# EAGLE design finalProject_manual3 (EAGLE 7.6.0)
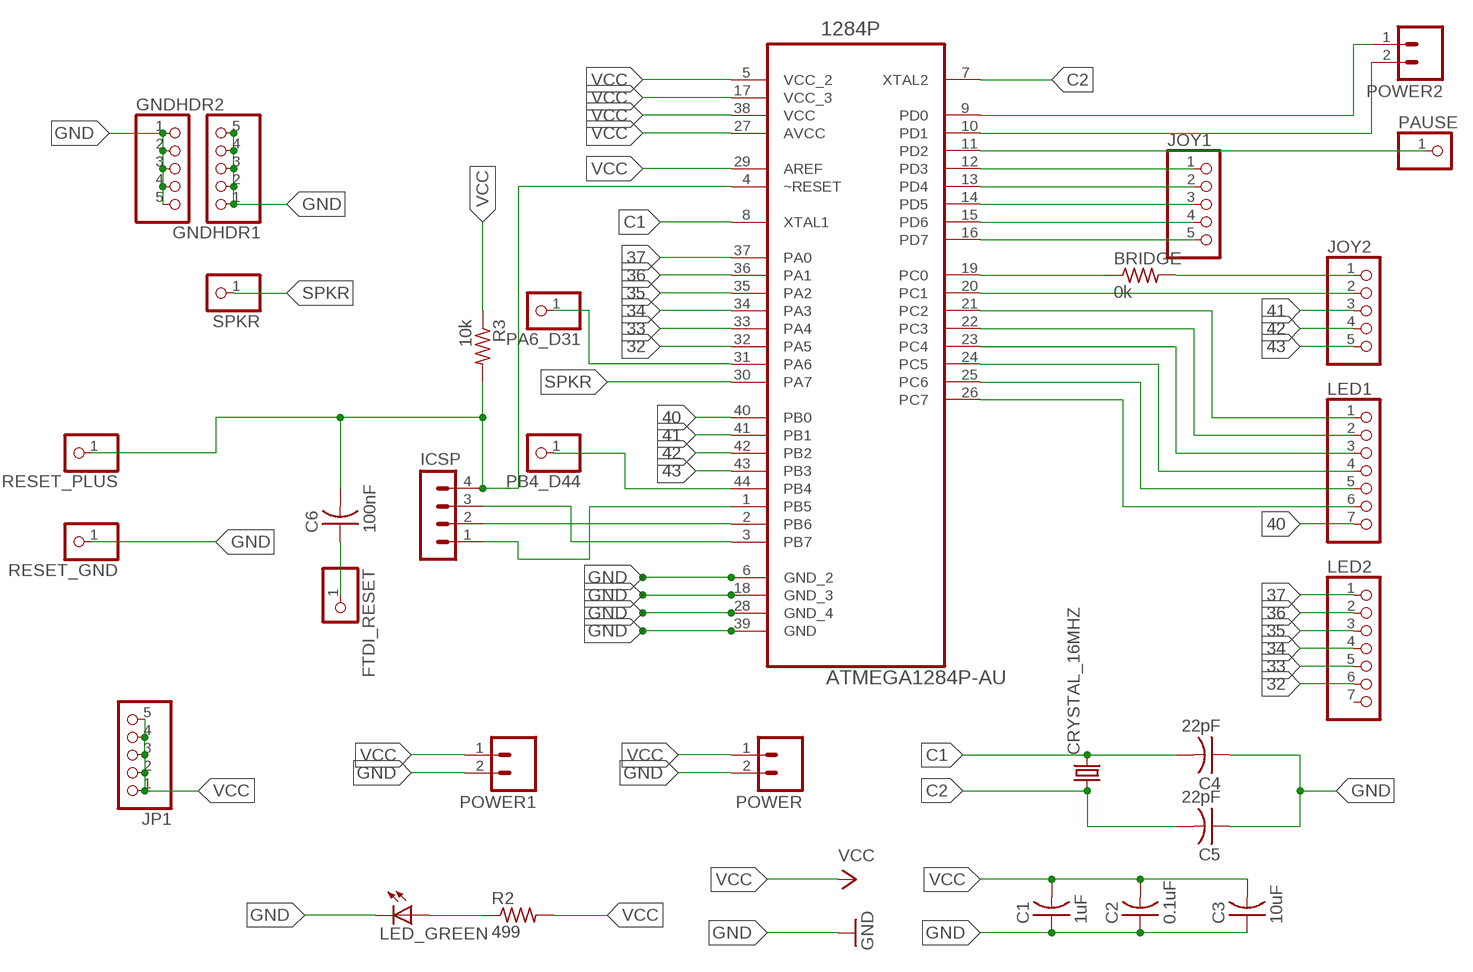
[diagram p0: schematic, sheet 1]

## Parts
1284P  ATMEGA1284P-AU  [QFP80P1200X1200X120-44N]
BRIDGE  0k  RES-US1206  [R1206]
C1  1uF  CAP-US1206  [C1206]
C2  0.1uF  CAP-US1206  [C1206]
C3  10uF  CAP-US1206  [C1206]
C4  22pF  CAP-US1206  [C1206]
C5  22pF  CAP-US1206  [C1206]
C6  100nF  CAP-US1206  [C1206]
CRYSTAL_16MHZ  CRYSTALHC49UP  [HC49UP]
FTDI_RESET  PINHD-1X1  [1X01]
GNDHDR1  PINHD-1X5  [1X05]
GNDHDR2  PINHD-1X5  [1X05]
ICSP  MA04-1  [MA04-1]
JOY1  PINHD-1X5  [1X05]
JOY2  PINHD-1X5  [1X05]
JP1  PINHD-1X5  [1X05]
LED1  PINHD-1X7  [1X07]
LED2  PINHD-1X7  [1X07]
LED_GREEN  LED1206  [1206]
PA6_D31  PINHD-1X1  [1X01]
PAUSE  PINHD-1X1  [1X01]
PB4_D44  PINHD-1X1  [1X01]
POWER  M02  [02P]
POWER1  M02  [02P]
POWER2  M02  [02P]
R2  499  RES-US1206  [R1206]
R3  10k  RES-US1206  [R1206]
RESET_GND  PINHD-1X1  [1X01]
RESET_PLUS  PINHD-1X1  [1X01]
SPKR  PINHD-1X1  [1X01]

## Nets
32: 1284P.32(PA5) LED2.6
33: 1284P.33(PA4) LED2.5
34: 1284P.34(PA3) LED2.4
35: 1284P.35(PA2) LED2.3
36: 1284P.36(PA1) LED2.2
37: 1284P.37(PA0) LED2.1
40: 1284P.40(PB0) LED1.7
41: 1284P.41(PB1) JOY2.3
42: 1284P.42(PB2) JOY2.4
43: 1284P.43(PB3) JOY2.5
C1: 1284P.8(XTAL1) C4.2 CRYSTAL_16MHZ.2
C2: 1284P.7(XTAL2) C5.2 CRYSTAL_16MHZ.1
GND: 1284P.6(GND_2) C1.1 C2.1 C3.1 C4.1 C5.1 GNDHDR1.1 GNDHDR1.2 GNDHDR1.3 GNDHDR1.4 GNDHDR1.5 GNDHDR2.1 GNDHDR2.2 GNDHDR2.3 GNDHDR2.4 GNDHDR2.5 LED_GREEN.2(C) POWER1.2 POWER.2 RESET_GND.1
N$1: 1284P.18(GND_3)
N$2: 1284P.28(GND_4)
N$3: 1284P.39(GND)
N$4: 1284P.19(PC0) BRIDGE.1
N$5: 1284P.44(PB4) PB4_D44.1
N$6: 1284P.20(PC1) JOY2.2
N$7: 1284P.16(PD7) JOY1.5
N$8: 1284P.14(PD5) JOY1.3
N$9: 1284P.13(PD4) JOY1.2
N$10: 1284P.12(PD3) JOY1.1
N$11: 1284P.11(PD2) PAUSE.1
N$12: 1284P.10(PD1) POWER2.2
N$13: 1284P.9(PD0) POWER2.1
N$14: 1284P.21(PC2) LED1.1
N$15: 1284P.22(PC3) LED1.2
N$16: 1284P.23(PC4) LED1.3
N$17: 1284P.24(PC5) LED1.4
N$18: 1284P.25(PC6) LED1.5
N$19: 1284P.26(PC7) LED1.6
N$20: 1284P.15(PD6) JOY1.4
N$21: 1284P.3(PB7) ICSP.3
N$22: 1284P.2(PB6) ICSP.2
N$23: 1284P.1(PB5) ICSP.1
N$24: BRIDGE.2 JOY2.1
N$26: LED_GREEN.1(A) R2.1
N$27: C6.1 FTDI_RESET.1
N$30: 1284P.31(PA6) PA6_D31.1
RESET_PLUS: 1284P.4(~RESET) C6.2 ICSP.4 R3.2 RESET_PLUS.1
SPKR: 1284P.30(PA7) SPKR.1
VCC: 1284P.5(VCC_2) 1284P.17(VCC_3) 1284P.27(AVCC) 1284P.29(AREF) 1284P.38(VCC) C1.2 C2.2 C3.2 JP1.1 JP1.2 JP1.3 JP1.4 JP1.5 POWER1.1 POWER.1 R2.2 R3.1
Unconnected: LED2.7

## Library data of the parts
1284P = 1284:ATMEGA1284P-AU: Microcontroller with Programmable Flash; MPN: ATMEGA1284P-AU; OC_FARNELL: 1715480; OC_NEWARK: 15R0263; PACKAGE: TQFP-44; SUPPLIER: Atmel
BRIDGE R2 R3 = fab:RES-US: Resistor (US Symbol)
C1-C6 = fab:CAP-US
CRYSTAL_16MHZ = crystal:CRYSTAL: CRYSTAL; OC_FARNELL: unknown; OC_NEWARK: unknown
FTDI_RESET PA6_D31 PAUSE PB4_D44 RESET_GND RESET_PLUS SPKR = pinhead:PINHD-1X1: PIN HEADER
GNDHDR1 GNDHDR2 JOY1 JOY2 JP1 = pinhead:PINHD-1X5: PIN HEADER
ICSP = con-lstb:MA04-1: PIN HEADER; OC_FARNELL: unknown; OC_NEWARK: unknown
LED1 LED2 = pinhead:PINHD-1X7: PIN HEADER
LED_GREEN = FAB_Hello:LED
POWER POWER1 POWER2 = con-amp-quick:M02: AMP QUICK CONNECTOR; OC_FARNELL: unknown; OC_NEWARK: unknown

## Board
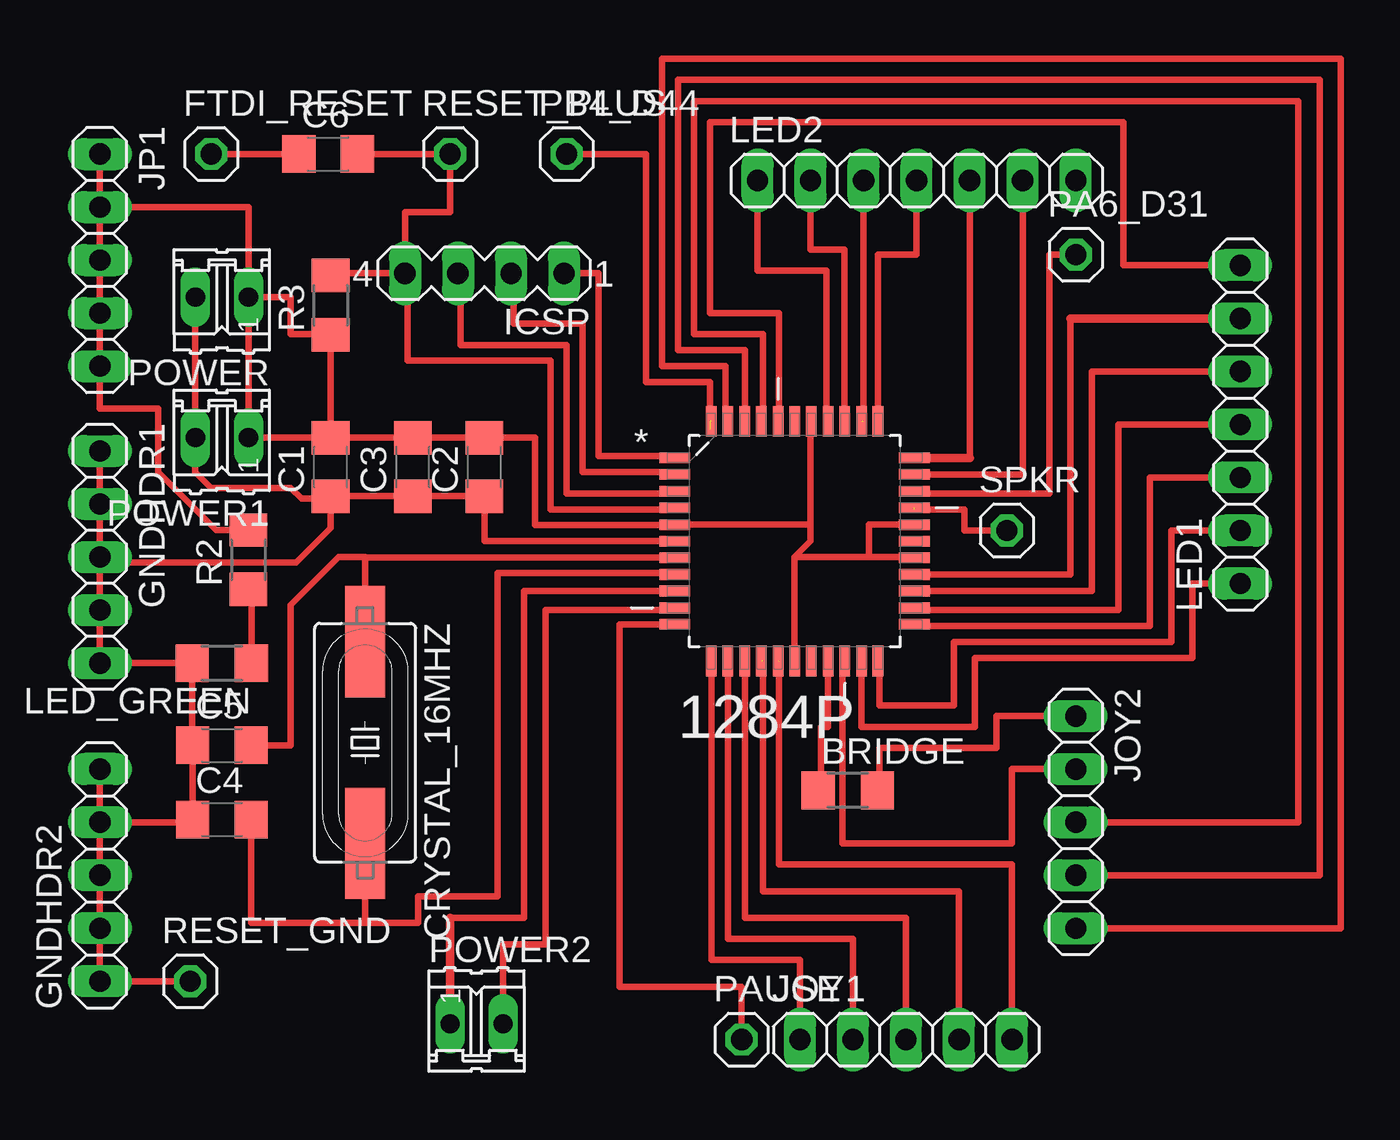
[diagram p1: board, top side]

No outline drawn. Coordinates in mm, seen from the top.
Copper layers (1*16): Top 0.035mm / dielectric 1.5mm / Bottom 0.035mm
Design rules "default": minimum track width 10mil, minimum drill 24mil, track to track 8mil, track to pad 8mil, pad to pad 8mil, via to via 8mil, smd to smd 8mil, copper to edge 40mil, drill to drill 8mil, minimum pad ring 10mil, minimum via ring 8mil, stop-mask expansion 4mil, vias tented up to drill 0mil, thermal gap 10mil

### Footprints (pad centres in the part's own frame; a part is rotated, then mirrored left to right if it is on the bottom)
QFP80P1200X1200X120-44N = smd 1.473 x 0.508: 1 -5.74,3.988; 2 -5.74,3.2; 3 -5.74,2.388; 4 -5.74,1.6; 5 -5.74,0.787; 6 -5.74,0; 7 -5.74,-0.787; 8 -5.74,-1.6; 9 -5.74,-2.388; 10 -5.74,-3.2; 11 -5.74,-3.988; 23 5.74,-3.988; 24 5.74,-3.2; 25 5.74,-2.388; 26 5.74,-1.6; 27 5.74,-0.787; 28 5.74,0; 29 5.74,0.787; 30 5.74,1.6; 31 5.74,2.388; 32 5.74,3.2; 33 5.74,3.988 | smd 0.508 x 1.473: 12 -3.988,-5.74; 13 -3.2,-5.74; 14 -2.388,-5.74; 15 -1.6,-5.74; 16 -0.787,-5.74; 17 0,-5.74; 18 0.787,-5.74; 19 1.6,-5.74; 20 2.388,-5.74; 21 3.2,-5.74; 22 3.988,-5.74; 34 3.988,5.74; 35 3.2,5.74; 36 2.388,5.74; 37 1.6,5.74; 38 0.787,5.74; 39 0,5.74; 40 -0.787,5.74; 41 -1.6,5.74; 42 -2.388,5.74; 43 -3.2,5.74; 44 -3.988,5.74
R1206 = smd 1.6 x 1.803: 1 -1.422,0; 2 1.422,0
C1206 = smd 1.6 x 1.8: 1 -1.4,0; 2 1.4,0
HC49UP = smd 5.334 x 1.93: 1 -4.826,0; 2 4.826,0
1X01 = drill 1.016 octagon: 1 0,0
1X05 = drill 1.016 long: 1 -5.08,0; 2 -2.54,0; 3 0,0; 4 2.54,0; 5 5.08,0
MA04-1 = drill 1.016 long: 1 -3.81,0; 2 -1.27,0; 3 1.27,0; 4 3.81,0
1X07 = drill 1.016 long: 1 -7.62,0; 2 -5.08,0; 3 -2.54,0; 4 0,0; 5 2.54,0; 6 5.08,0; 7 7.62,0
1206 = smd 1.6 x 1.803: 1 -1.422,0; 2 1.422,0
02P = drill 0.914 long: 1 -1.27,0; 2 1.27,0

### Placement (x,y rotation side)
1284P  33.27,46.23 0 top
BRIDGE  35.81,34.29 0 top
C1  11.05,49.78 90 top
C2  18.41,49.78 90 top
C3  14.99,49.78 90 top
C4  5.84,32.89 0 top
C5  5.84,36.45 0 top
C6  10.92,64.77 0 top
CRYSTAL_16MHZ  12.7,36.58 270 top
FTDI_RESET  5.33,64.77 0 top
GNDHDR1  0,45.47 270 top
GNDHDR2  0,30.23 90 top
ICSP  18.41,59.05 180 top
JOY1  38.61,22.35 0 top
JOY2  46.74,32.77 270 top
JP1  0,59.69 270 top
LED1  54.61,51.82 90 top
LED2  39.12,63.5 0 top
LED_GREEN  5.84,40.39 180 top
PA6_D31  46.74,59.94 0 top
PAUSE  30.73,22.35 0 top
PB4_D44  22.35,64.77 0 top
POWER  5.84,57.91 180 top
POWER1  5.84,51.18 180 top
POWER2  18.03,23.11 0 top
R2  7.11,45.34 90 top
R3  11.05,57.53 90 top
RESET_GND  4.32,25.15 0 top
RESET_PLUS  16.76,64.77 0 top
SPKR  43.43,46.74 0 top

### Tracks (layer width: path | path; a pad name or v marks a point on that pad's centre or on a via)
32
  Top 0.305: 1284P.32 44.2,49.43 LED2.6
33
  Top 0.305: 41.66,50.22 LED2.5
  Top 0.406: 1284P.33 41.66,50.22
34
  Top 0.305: LED2.4 39.12,59.94 37.26,59.94 1284P.34
35  (1 unrouted)
  Top 0.305: 36.58,51.97 LED2.3
36
  Top 0.305: 1284P.36 35.66,60.2 34.04,60.2 LED2.2
37
  Top 0.305: 1284P.37 34.8,51.97 34.8,59.18 31.5,59.18 LED2.1
40
  Top 0.305: 32.51,51.97 32.51,57.15 29.21,57.15 29.21,66.29 49.02,66.29 49.02,59.44 LED1.7
  Top 0.406: 1284P.40 32.51,51.97
41
  Top 0.305: JOY2.3 57.4,32.77 57.4,67.06 57.4,67.31 28.45,67.31 28.45,56.13 31.75,56.13 31.75,51.97 1284P.41
42
  Top 0.305: JOY2.4 58.42,30.23 58.42,68.33 27.69,68.33 27.69,55.37 30.89,55.37 1284P.42
43
  Top 0.305: 1284P.43 29.97,51.97 29.97,54.61 26.92,54.61 26.92,69.34 59.44,69.34 59.44,69.09 59.44,68.83 59.44,27.69 JOY2.5
C1
  Top 0.305: 1284P.8 27.53,44.7 19.05,44.7 19.05,29.21 15.24,29.21 15.24,27.94 12.7,27.94 | 12.7,27.94 7.24,27.94 C4.2 | CRYSTAL_16MHZ.2 12.7,27.94
C2
  Top 0.305: 1284P.7 12.7,45.44 | 12.7,45.44 CRYSTAL_16MHZ.1 | C5.2 9.14,36.45 9.14,43.18 11.43,45.47 12.68,45.47 12.7,45.44 | 12.7,45.47 12.7,45.44
GND
  Top 0.305: 18.54,48.38 C2.1 | C2.1 C3.1 C1.1 | GNDHDR2.5 GNDHDR2.4 | GNDHDR2.4 GNDHDR2.3 GNDHDR2.2 GNDHDR2.1 RESET_GND.1 | GNDHDR1.1 GNDHDR1.2 GNDHDR1.3 | GNDHDR1.3 GNDHDR1.4 GNDHDR1.5 LED_GREEN.2 4.42,36.45 C5.1 C4.1 4.44,32.77 GNDHDR2.4 | POWER.2 POWER1.2 4.57,49.53 5.33,48.77 9.14,48.77 9.65,48.26 10.93,48.26 C1.1 | 1284P.6 18.41,46.23 C2.1 | C1.1 11.05,46.86 9.4,45.21 0.25,45.21 GNDHDR1.3
N$4
  Top 0.305: BRIDGE.1 34.54,34.29 34.54,37.34 34.87,37.34 1284P.19
N$5  (2 unrouted)
  Top 0.305: PB4_D44.1 26.16,64.77 26.16,53.85 29.21,53.85 29.21,51.97
N$6
  Top 0.305: 1284P.20 35.56,40.49 35.56,31.75 43.69,31.75 43.69,35.31 JOY2.2
N$7  (1 unrouted)
  Top 0.305: 32.51,40.49 32.51,30.73 43.69,30.73 JOY1.5
N$8
  Top 0.305: 1284P.14 30.89,28.19 38.61,28.19 JOY1.3
N$9
  Top 0.305: 1284P.13 30.07,27.18 36.07,27.18 JOY1.2
N$10
  Top 0.305: JOY1.1 33.53,26.16 29.72,26.16 29.46,26.16 29.29,26.16 1284P.12
N$11
  Top 0.305: 1284P.11 24.89,42.24 24.89,24.89 30.73,24.89 PAUSE.1
N$12
  Top 0.305: POWER2.2 19.3,26.92 21.34,26.92 21.34,42.93 27.69,42.93 27.69,43.03
  Top 0.406: 1284P.10 27.69,43.03
N$13
  Top 0.305: 1284P.9 20.32,43.84 20.32,28.19 16.76,28.19
  Top 0.406: 16.76,28.19 POWER2.1
N$14
  Top 0.305: 1284P.21 36.47,37.34 41.91,37.34 41.91,40.64 52.32,40.64 52.32,44.2 LED1.1
N$15
  Top 0.305: LED1.2 51.31,46.74 51.31,41.4 40.89,41.4 40.89,38.35 37.34,38.35 37.34,40.49 1284P.22
N$16
  Top 0.305: LED1.3 50.29,49.28 50.29,42.16 39.01,42.16 1284P.23
N$17
  Top 0.305: LED1.4 48.77,51.82 48.77,43.18 48.77,42.93 39.12,42.93 39.12,43.03 1284P.24
N$18
  Top 0.305: 1284P.25 47.5,43.84 47.5,54.36 LED1.5
N$19
  Top 0.305: 1284P.26 46.48,44.63 46.48,56.9
  Top 0.406: 46.48,56.9 LED1.6
N$20  (1 unrouted)
  Top 0.305: JOY1.4 41.15,29.46 32.51,29.46 31.75,29.46 31.75,40.49
N$21
  Top 0.305: 1284P.3 27.53,48.51 22.35,48.51 22.35,55.63 17.27,55.63 17.27,59.05 ICSP.3
N$22
  Top 0.305: 1284P.2 27.53,49.53 23.11,49.53 23.11,56.64 19.81,56.64 19.81,59.05 ICSP.2
N$23
  Top 0.305: 1284P.1 27.53,50.29 23.88,50.29 23.88,59.05 ICSP.1
N$24
  Top 0.305: BRIDGE.2 37.34,34.29 37.34,36.32 42.93,36.32 42.93,37.85 JOY2.1
N$26
  Top 0.305: R2.1 7.26,43.92 LED_GREEN.1
N$27
  Top 0.305: C6.1 FTDI_RESET.1
N$30
  Top 0.305: 1284P.31 39.01,48.51 45.47,48.51 45.47,59.94 PA6_D31.1
RESET_PLUS
  Top 0.305: 1284P.4 27.53,47.75 21.59,47.75 21.59,54.86 14.73,54.86 14.73,59.05 ICSP.4 | ICSP.4 14.61,61.98 16.76,61.98 RESET_PLUS.1 C6.2 | R3.2 11.05,59.05 ICSP.4
SPKR  (1 unrouted)
  Top 0.305: SPKR.1 41.4,46.74 41.4,47.75 39.01,47.75
VCC
  Top 0.305: 1284P.17 33.27,45.47 | 33.27,45.47 36.83,45.47 | 36.83,45.47 39.01,45.47 | 1284P.29 36.83,47.02 36.83,45.47 | 34.04,47.02 1284P.5 27.53,46.99 20.83,46.99 20.83,51.18 C2.2 C3.2 C1.2 | POWER.1 9.14,57.91 9.14,56.13 11.05,56.13 R3.1 C1.2 | POWER.1 7.11,62.23 JP1.2 | JP1.1 JP1.2 | JP1.2 JP1.3 JP1.4 JP1.5 | JP1.5 JP1.2 | POWER.1 POWER1.1 C1.2 | 34.04,51.97 34.04,47.02 | 34.04,47.02 34.04,46.23 33.27,45.47 | JP1.5 0,52.58 2.79,52.58 2.79,49.53 5.56,46.76 R2.2
  Top 0.406: 39.01,45.47 1284P.27 | 1284P.38 34.04,51.97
